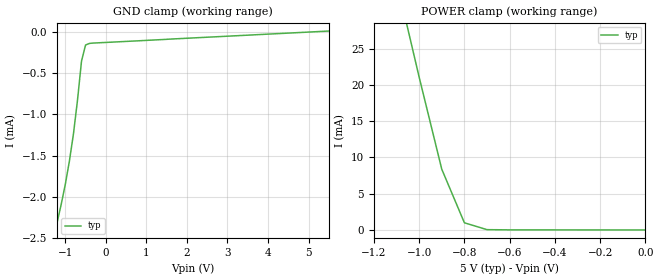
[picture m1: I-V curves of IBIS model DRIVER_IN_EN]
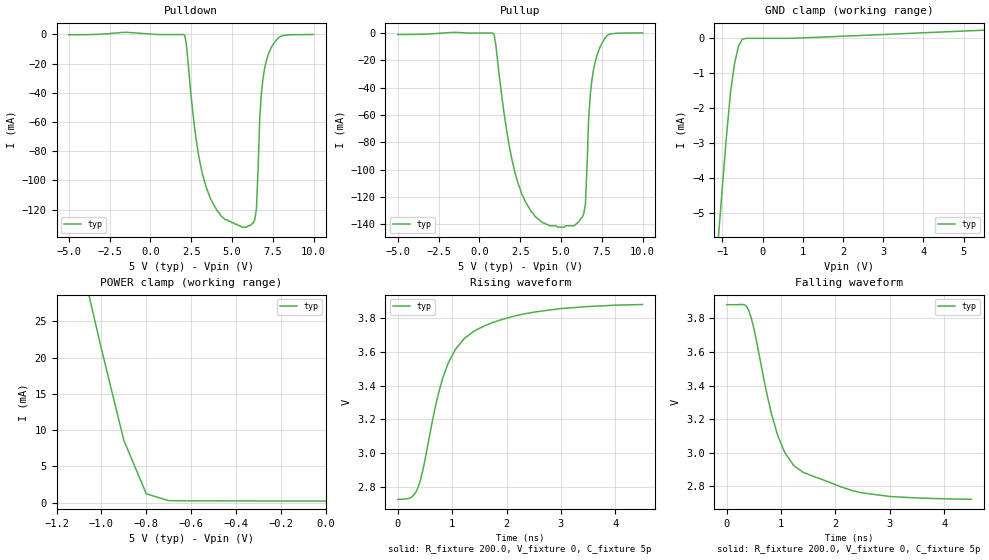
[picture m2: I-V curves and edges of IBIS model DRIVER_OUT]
|   Texas Instruments Incorporated
|   Data Transmissions Products
|   IBIS Model for TB5D1M
|   16DW SOIC Package
[IBIS Ver]   3.2
[Comment char]   |_char
[File name]   tb5d1m.ibs
[File Rev]   1.0
[Date]   14Apr03
[Source]   File originated at Texas Instruments Incorporated.
   Data Transmission Products Group. All data based on
   Simulation.
[Notes]
[Disclaimer]
(C) Copyright Texas Instruments Incorporated 2003
   All rights reserved
  Texas Instruments Incorporated hereby grants the user of this IBIS
model a non-exclusive, nontransferable license to use this IBIS model
under the following terms.  Before using this IBIS model, the user
should read this license.  If the user does not accept these terms,
the IBIS model should be returned to Texas Instruments within 30 days.
  The user is granted this license only to use the IBIS model and
is not granted rights to sell, load, rent, lease or license the IBIS
model in whole or in part, or in modified form to anyone other than
user.  User may modify the IBIS model to suit its specific applications
but rights to derivative works and such modifications shall belong to
Texas Instruments.
  This IBIS model is provided on an "AS IS" basis and Texas Instruments
makes absolutely no warranty with respect to the information contained
herein.  TEXAS INSTRUMENTS DISCLAIMS AND CUSTOMER WAIVES ALL WARRANTIES,
EXPRESS OR IMPLIED, INCLUDING WARRANTIES OF MERCHANTABILITY OR FITNESS
FOR A PARTICULAR PURPOSE. The entire risk as to quality and performance
is with the Customer. ACCORDINGLY, IN NO EVENT SHALL THE COMPANY BE LIABLE
FOR ANY DAMAGES, WHETHER IN CONTRACT OR TORT,INCLUDING ANY LOST PROFITS
OR OTHER INCIDENTAL, CONSEQUENTIAL, EXEMPLARY, OR PUNITIVE DAMAGES ARISING
OUT OF THE USE OR APPLICATION OF THE IBIS model provided in this package.
Further, Texas Instruments reserves the right to discontinue or make changes
without notice to any product herein to improve reliability, function, or
design. Texas Instruments does not convey any license under patent rights
or any other intellectual property rights, including those of third parties.
Contact Texas Instruments at ATTN:DATA TRANSMISSIONS
[Copyright]   Copyright 2003, Texas Instruments, All Rights Reserved
[Component]   TB5D1M
[Manufacturer]  Texas Instruments
[Package]
|   typ   min   max
R_pkg   0.046   0.034   0.057
L_pkg   4.858nH   3.987nH   6.214nH
C_pkg   0.715pF   0.502pF   1.046pF
[Pin]   signal_name   model_name   R_pin   L_pin   C_pin
1   AI   DRIVER_IN_EN   0.057   6.214nH   1.026pF
2   AO   DRIVER_OUT   0.055   5.236nH   0.818pF
3   AO(-)   DRIVER_OUT   0.034   3.987nH   0.723pF
4   E1   DRIVER_IN_EN   0.036   3.996nH   0.726pF
5   BO(-)   DRIVER_OUT   0.036   3.996nH   0.726pF
6   BO   DRIVER_OUT   0.034   3.987nH   0.704pF
7   BI   DRIVER_IN_EN   0.055   5.236nH   0.818pF
8   GND   GND   0.057   6.214nH   1.046pF
9   CI   DRIVER_IN_EN   0.057   6.214nH   0.827pF
10   CO   DRIVER_OUT   0.055   5.236nH   0.597pF
11   CO(-)   DRIVER_OUT   0.034   3.987nH   0.502pF
12   E2   DRIVER_IN_EN   0.036   3.996nH   0.505pF
13   DO(-)   DRIVER_OUT   0.036   3.996nH   0.505pF
14   DO   DRIVER_OUT   0.034   3.987nH   0.502pF
15   DI   DRIVER_IN_EN   0.055   5.236nH   0.597pF
16   VCC   POWER   0.057   6.214nH   0.827pF
[Diff_pin]   inv_pin   vdiff   tdelay_typ   tdelay_min   tdelay_max
| The 'AO(+) (or 'xO(+)')' and inv_pins, 'AO(-) (or 'xO(-)')', pins
| are Diff_pins
   2   3   0   0   0   0
   6   5   0   0   0   0
   10   11   0   0   0   0
   14   13   0   0   0   0
| Models and submodels in the file (2): DRIVER_IN_EN (Input), DRIVER_OUT (Output_ECL)
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|   Driver Input Model
[Model]   DRIVER_IN_EN
Model_type   Input
|Signals   AI,BI,CI,DI,E1,E2
Vinh = 2.4
Vinl = 0.4
|   typ   min   max
C_comp   979fF   NA   NA
|   typ   min   max
[Temperature Range]   25.0   NA   NA
[Voltage range]   5.0V   NA   NA
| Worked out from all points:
|   GND clamp passes 1 mA (typ) near -0.74 V on its own axis
|   POWER clamp passes 1 mA (typ) near -0.80 V on its own axis
[GND_clamp]
| Voltage   I(typ)   I(min)   I(max)
-5.5V     -10.4mA    NA         NA
-1.3V     -2.52mA    NA         NA
-1.2V     -2.31mA    NA         NA
-1.1V     -2.09mA    NA         NA
-1V       -1.85mA    NA         NA
-900mV    -1.57mA    NA         NA
-800mV    -1.24mA    NA         NA
-700mV    -830uA     NA         NA
-600mV    -351uA     NA         NA
-500mV    -156uA     NA         NA
-300mV    -132uA     NA         NA
5.5V      13.7uA     NA         NA
[Power_clamp]
| Note that the[POWER_clamp]voltage table is referenced to Vcc
| and is calculated using Vtable=Vcc - Vmeasured.
|   Voltage   I(typ)   I(min)   I(max)
-5V       163mA      NA         NA
-1.1V     34.4mA     NA         NA
-1V       21.1mA     NA         NA
-900mV    8.39mA     NA         NA
-800mV    993uA      NA         NA
-700mV    43.9uA     NA         NA
0V        1.12uA     NA         NA
|   Driver Output Model
[Model]   DRIVER_OUT
|Model_type   3-state_ECL
Model_type   Output_ECL
| Signals   O(+),O(-)
Vmeas = 3.2V   |Reference voltage for timing measurements
Cref = 5pF   |Timing specification test load capacitance value
Rref = 200   |Note: 200 Ohm load; single ended configuration
| variable   typ   min   max
C_comp   583fF   NA   NA
|   typ   min   max
[Temperature Range]   25.0   NA   NA
[Voltage range]   5.0V   NA   NA
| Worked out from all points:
|   GND clamp passes 1 mA (typ) near -0.73 V on its own axis
|   POWER clamp passes 1 mA (typ) near -0.78 V on its own axis
|   rising waveform, R_fixture 200.0, V_fixture 0, C_fixture 5p: 20-80 % time 649ps typ, NA min, NA max; typ from 2.73 V to 3.88 V
|   falling waveform, R_fixture 200.0, V_fixture 0, C_fixture 5p: 20-80 % time 610ps typ, NA min, NA max; typ from 3.88 V to 2.72 V
[Pulldown]
|   Voltage   I(typ)   I(min)   I(max)
-5V       -300uA     NA         NA
2.1V      -574uA     NA         NA
2.8V      -71.6mA    NA         NA
3.4V      -104mA     NA         NA
4.3V      -124mA     NA         NA
5.9V      -132mA     NA         NA
6.5V      -119mA     NA         NA
6.7V      -57.6mA    NA         NA
6.8V      -40.6mA    NA         NA
7.2V      -14.5mA    NA         NA
8V        -1.3mA     NA         NA
10V       -100uA     NA         NA
[Pullup]
|   Voltage   I(typ)   I(min)   I(max)
| Note that the[Pullup]voltage table is referenced to Vcc
| and is calculated using Vtable=Vcc - Vmeasured.
-5V       -1.3mA     NA         NA
900mV     -1.15mA    NA         NA
1.8V      -80.4mA    NA         NA
2.6V      -118mA     NA         NA
3.9V      -139mA     NA         NA
5.2V      -142mA     NA         NA
6.4V      -132mA     NA         NA
6.5V      -125mA     NA         NA
6.7V      -62.2mA    NA         NA
6.8V      -44.8mA    NA         NA
7.4V      -10.4mA    NA         NA
10V       -100uA     NA         NA
[GND_clamp]
|   Voltage   I(typ)   I(min)   I(max)
| Outputs in High Impedance (off)
-5.5V     -173mA     NA         NA
-1.1V     -5.68mA    NA         NA
-1V       -4.2mA     NA         NA
-900mV    -2.79mA    NA         NA
-800mV    -1.54mA    NA         NA
-700mV    -719uA     NA         NA
-600mV    -212uA     NA         NA
-500mV    -19.1uA    NA         NA
900mV     8.68uA     NA         NA
5.5V      232uA      NA         NA
[Power_clamp]
| Note that the[POWER_clamp]voltage table is referenced to Vcc
| and is calculated using Vtable=Vcc - Vmeasured.
|   Voltage   I(typ)   I(min)   I(max)
-5V       167mA      NA         NA
-1.1V     34.5mA     NA         NA
-1V       21.2mA     NA         NA
-900mV    8.58mA     NA         NA
-800mV    1.21mA     NA         NA
-700mV    267uA      NA         NA
0V        208uA      NA         NA
[Ramp]
|   typ   min   max
dV/dt_r   0.694/659ps   NA   NA
dV/dt_f   0.695/611ps   NA   NA
R_load = 200ohm
[Rising Waveform]
R_fixture = 200.0
V_fixture = 0
C_fixture = 5p
|   V(typ)   V(min)   V(max)
0s        2.729V     NA         NA
250ps     2.741V     NA         NA
375ps     2.801V     NA         NA
450ps     2.885V     NA         NA
825ps     3.442V     NA         NA
1.05ns    3.607V     NA         NA
1.225ns   3.678V     NA         NA
1.7ns     3.766V     NA         NA
2.325ns   3.823V     NA         NA
4.5ns     3.878V     NA         NA
[Falling Waveform]
R_fixture = 200.0
V_fixture = 0
C_fixture = 5p
|   V(typ)   V(min)   V(max)
0s        3.882V     NA         NA
300ps     3.883V     NA         NA
400ps     3.85V      NA         NA
500ps     3.739V     NA         NA
750ps     3.335V     NA         NA
925ps     3.117V     NA         NA
1.075ns   2.998V     NA         NA
1.25ns    2.92V      NA         NA
2.45ns    2.764V     NA         NA
4.5ns     2.723V     NA         NA
